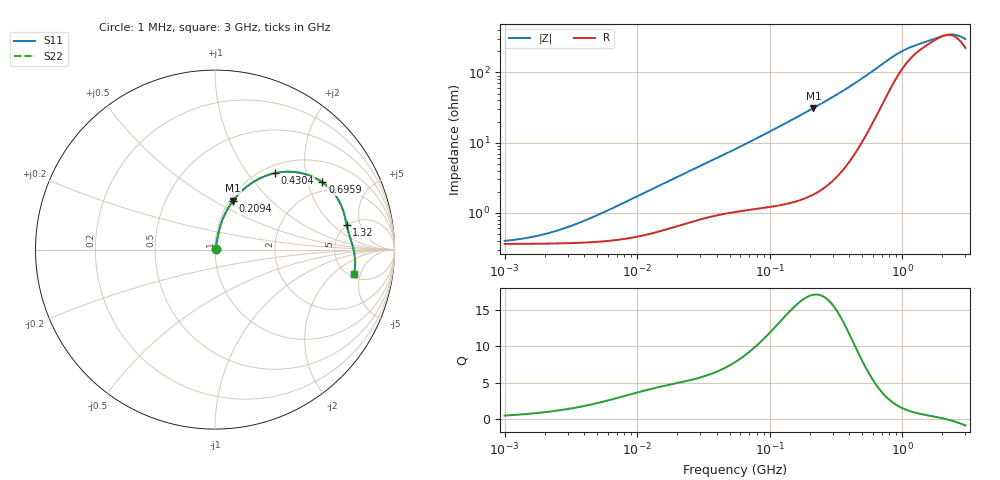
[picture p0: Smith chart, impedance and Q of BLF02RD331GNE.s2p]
! BLF02RD331GNE
# Hz S RI R 50
!Freq.(Hz) S11(Real) S11(Imag) S21(Real) S21(Imag) S12(Real) S12(Imag) S22(Real) S22(Imag)
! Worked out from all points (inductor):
!   401 points, 1 MHz to 3 GHz, reference 50 ohm
!   read as one part in series: L = 26.5 nH near 7.55 MHz
!   highest Q = 17 at 213.6 MHz (marker M1), where L = 23.1 nH
!   self-resonance near 2.129 GHz
!   S11 on the Smith chart (normalised r, x): 1 MHz: 1.01, +0.00; 209.4 MHz: 1.04, +0.61; 430.4 MHz: 1.13, +1.36; 695.9 MHz: 1.66, +2.48; 1.32 GHz: 4.97, +3.05; 3 GHz: 5.47, -3.94
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1000000  0.0036 0.00168  0.9964 -0.00168  0.9964 -0.00168  0.0036 0.00168
1405328  0.00361 0.00236  0.9964 -0.00236  0.9964 -0.00236  0.00361 0.00236
1974946  0.00364 0.00332  0.9964 -0.00332  0.9964 -0.00332  0.00364 0.00332
2720446  0.00369 0.00457  0.9963 -0.00457  0.9963 -0.00457  0.00369 0.00457
3823119  0.00379 0.00641  0.9962 -0.00641  0.9962 -0.00641  0.00379 0.00641
6180806  0.00409 0.0103  0.9959 -0.0103  0.9959 -0.0103  0.00409 0.0103
1.461624e7  0.00596 0.0235  0.994 -0.0235  0.994 -0.0235  0.00596 0.0235
5.477226e7  0.0163 0.0779  0.9837 -0.0779  0.9837 -0.0779  0.0163 0.0779
1.103592e8  0.0357 0.1502  0.9643 -0.1502  0.9643 -0.1502  0.0357 0.1502
2.094008e8  0.0977 0.2689  0.9023 -0.2689  0.9023 -0.2689  0.0977 0.2689
2.136344e8  0.1011 0.2735  0.8989 -0.2735  0.8989 -0.2735  0.1011 0.2735
3.062963e8  0.1892 0.3605  0.8108 -0.3605  0.8108 -0.3605  0.1892 0.3605
4.304467e8  0.3332 0.4257  0.6668 -0.4257  0.6668 -0.4257  0.3332 0.4257
5.473095e8  0.4677 0.4289  0.5323 -0.4289  0.5323 -0.4289  0.4677 0.4289
6.958997e8  0.5985 0.375  0.4015 -0.375  0.4015 -0.375  0.5985 0.375
8.005644e8  0.6563 0.3217  0.3437 -0.3217  0.3437 -0.3217  0.6563 0.3217
9.779672e8  0.706 0.2381  0.294 -0.2381  0.294 -0.2381  0.706 0.2381
1.320433e9  0.7344 0.1355  0.2656 -0.1355  0.2656 -0.1355  0.7344 0.1355
1.931433e9  0.7643 0.0312  0.2357 -0.0312  0.2357 -0.0312  0.7643 0.0312
2.221924e9  0.7752 -0.0149  0.2248 0.0149  0.2248 0.0149  0.7752 -0.0149
2.556106e9  0.7806 -0.0685  0.2194 0.0685  0.2194 0.0685  0.7806 -0.0685
3e9  0.7746 -0.1374  0.2254 0.1374  0.2254 0.1374  0.7746 -0.1374
